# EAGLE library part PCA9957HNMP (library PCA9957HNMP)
LED Lighting Drivers I2C 5 V Constant Current LED Controller Source: Datasheet
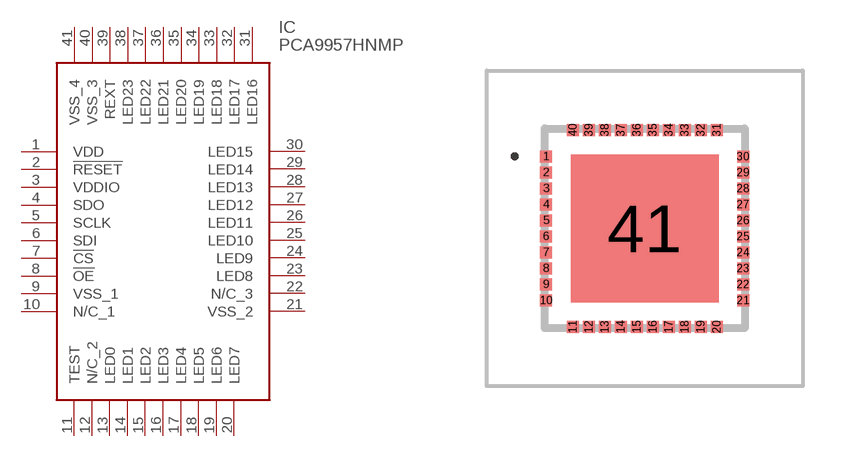
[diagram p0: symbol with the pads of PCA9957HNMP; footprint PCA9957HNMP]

Designator prefix IC

## PCA9957HNMP (Description: LED Lighting Drivers I2C 5 V Constant Current LED Controller; Height: 1mm; Manufacturer_Name: NXP; Manufacturer_Part_Number: PCA9957HNMP)  [PCA9957HNMP]
1  VDD
2  !RESET
3  VDDIO
4  SDO
5  SCLK
6  SDI
7  !CS
8  !OE
9  VSS_1
10  N/C_1
11  TEST
12  N/C_2
13  LED0
14  LED1
15  LED2
16  LED3
17  LED4
18  LED5
19  LED6
20  LED7
21  VSS_2
22  N/C_3
23  LED8
24  LED9
25  LED10
26  LED11
27  LED12
28  LED13
29  LED14
30  LED15
31  LED16
32  LED17
33  LED18
34  LED19
35  LED20
36  LED21
37  LED22
38  LED23
39  REXT
40  VSS_3
41  VSS_4

## Footprint PCA9957HNMP (pad centres in mm)
PCA9957HNMP-10
smd 0.3 x 0.3: 1 -2.463,1.8; 2 -2.463,1.4; 3 -2.463,1; 4 -2.463,0.6; 5 -2.463,0.2; 6 -2.463,-0.2; 7 -2.463,-0.6; 8 -2.463,-1; 9 -2.463,-1.4; 10 -2.463,-1.8; 11 -1.8,-2.463; 12 -1.4,-2.463; 13 -1,-2.463; 14 -0.6,-2.463; 15 -0.2,-2.463; 16 0.2,-2.463; 17 0.6,-2.463; 18 1,-2.463; 19 1.4,-2.463; 20 1.8,-2.463; 21 2.463,-1.8; 22 2.463,-1.4; 23 2.463,-1; 24 2.463,-0.6; 25 2.463,-0.2; 26 2.463,0.2; 27 2.463,0.6; 28 2.463,1; 29 2.463,1.4; 30 2.463,1.8; 31 1.8,2.463; 32 1.4,2.463; 33 1,2.463; 34 0.6,2.463; 35 0.2,2.463; 36 -0.2,2.463; 37 -0.6,2.463; 38 -1,2.463; 39 -1.4,2.463; 40 -1.8,2.463
smd 3.7 x 3.7: 41 0,0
